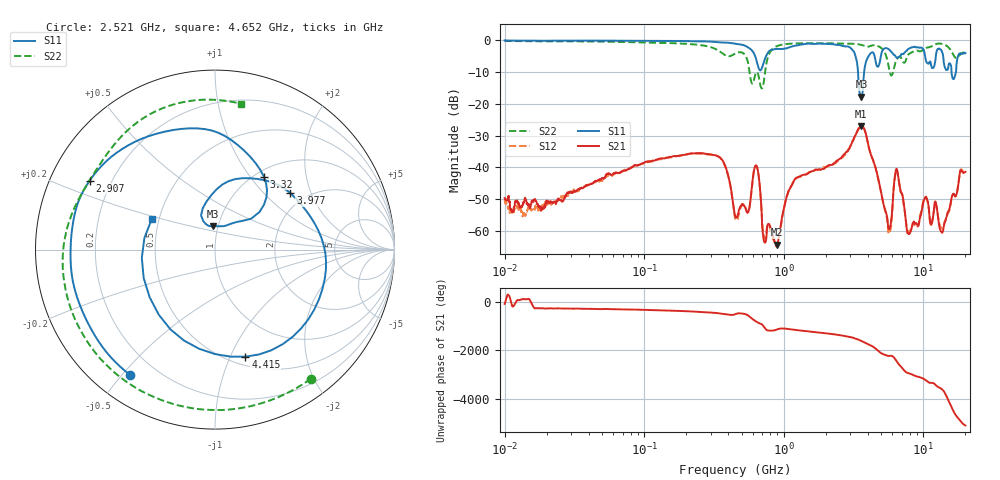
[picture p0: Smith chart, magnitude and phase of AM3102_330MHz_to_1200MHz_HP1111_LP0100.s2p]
! Date/Time: Tue, Sep 11, 2018 5:24 PM
! Network Analyzer: Agilent Technologies E8362B Rev: A.07.50.63
! Sweep from 0.010 to 20.000 GHz, 1601 Points, Sweep Type: LOG
! Power Supply: 4.949 V, 0.001 A
# Hz S DB R 50
!freq MagS11 AngS11 MagS21 AngS21 MagS12 AngS12 MagS22 AngS22
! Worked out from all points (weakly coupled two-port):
!   1601 points, 10 MHz to 20 GHz, reference 50 ohm
!   highest |S21| = -27.10 dB at 3.565 GHz (marker M1); lowest = -64.4 dB at 890.6 MHz (marker M2)
!   lowest |S11| = -17.7 dB at 3.599 GHz (marker M3), VSWR 1.30, Z = 47.3 + j12.4 ohm
!   |S11| at or under -10 dB: 3.402 GHz to 3.763 GHz (361.3 MHz wide, 10.1 % of centre); 15.91 GHz to 17.11 GHz (1.205 GHz wide, 7.3 % of centre)
!   |S22| runs from -15.1 to -0.1 dB; largest |S21 - S12| = 0.0058
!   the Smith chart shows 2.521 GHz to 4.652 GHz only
!   S11 on the Smith chart (normalised r, x): 2.521 GHz: 0.11, -0.52; 2.907 GHz: 0.12, +0.25; 3.32 GHz: 1.09, +1.17; 3.977 GHz: 1.67, +1.44; 4.415 GHz: 0.59, -1.14; 4.652 GHz: 0.46, +0.18
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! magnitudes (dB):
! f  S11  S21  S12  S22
! 10 MHz  0.0  -49.7  -50.5  -0.1
! 35.55 MHz  -0.1  -46.5  -46.4  -0.3
! 126.4 MHz  -0.2  -37.5  -37.5  -0.7
! 342.8 MHz  -0.6  -36.7  -36.7  -3.3
! 447.2 MHz  -1.0  -55.2  -55.9  -4.2
! 632.6 MHz  -5.8  -39.4  -39.5  -10.1
! 726 MHz  -6.3  -63.7  -62.4  -11.7
! 890.6 MHz  -2.7  -64.4  -64.6  -1.8
! 1.59 GHz  -1.1  -41.3  -41.2  -0.9
! 2.521 GHz  -1.5  -37.3  -37.4  -1.0
! 2.907 GHz  -2.0  -34.5  -34.3  -1.0
! 3.32 GHz  -6.2  -29.2  -29.2  -1.1
! 3.565 GHz  -17.7  -27.1  -27.0  -1.4
! 3.599 GHz  -17.7  -27.2  -27.0  -1.4
! 3.977 GHz  -5.6  -31.8  -31.7  -2.0
! 4.415 GHz  -4.1  -38.5  -38.4  -1.5
! 4.652 GHz  -8.2  -41.9  -42.0  -1.7
! 5.652 GHz  -2.7  -59.4  -60.9  -8.4
! 6.426 GHz  -5.4  -40.5  -40.8  -6.1
! 7.882 GHz  -2.6  -61.1  -60.3  -4.3
! 13.61 GHz  -3.6  -60.7  -59.3  -1.1
! 20 GHz  -4.0  -41.5  -42.0  -3.8
